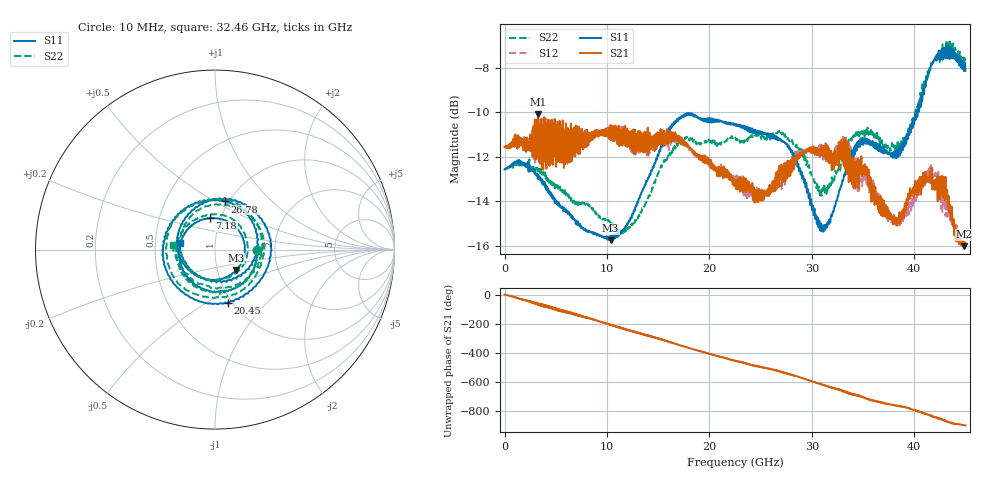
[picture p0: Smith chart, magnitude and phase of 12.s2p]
! 9/19/2025 2:51:32 PM
! C:\USERS\VECTORSTARUSER\DESKTOP\1942\12.S2P
! CHANNEL.1
! TR.MEASUREMENT
! CORRECTED.DATA
! RF.CORRECTION: FULL.TWO.PORT.CAL.PORT.1.2
! AVERAGING.OFF
! IF.BANDWIDTH: 1KHZ
! SWEEPTYPE:  FREQ.SWEEP(Linear)
! Reference Plane Port Info
! PORT:  PORT1  PORT2
! DISTANCE:  0  m  0  m
! TIME:  0  s  0  s
! PHASE.OFFSET:  0 °  0 °
! LOSS:  0  dB  0  dB
! REF.LOSS:  0  dB  0  dB
! REF.FREQ:  0  Hz  0  Hz
! Power Info
! POWER:  -10  dBm  -10  dBm
! EFF.POWER:  -10  dBm  -10  dBm
! SOURCE.ATTEN:  0  dB  0  dB
! TEST.ATTEN:  0  dB  0  dB
# GHZ S RI R 50.0
! FREQ.GHZ  S11RE  S11IM  S21RE  S21IM  S12RE  S12IM  S22RE  S22IM
!; PortSelection: Port_12
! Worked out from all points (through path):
!   1601 points, 10 MHz to 45 GHz, reference 50 ohm
!   highest |S21| = -10.10 dB at 3.272 GHz (marker M1); lowest = -16.0 dB at 44.86 GHz (marker M2)
!   group delay of S21, straight-line fit = 55.4 ps
!   lowest |S11| = -15.8 dB at 10.36 GHz (marker M3), VSWR 1.39, Z = 61.3 - j14.3 ohm
!   |S11| at or under -10 dB: start of sweep to 40.21 GHz; 40.25848 GHz to 40.34143 GHz (82.95 MHz wide, 0.206 % of centre)
!   |S22| runs from -15.5 to -6.8 dB; largest |S21 - S12| = 0.072
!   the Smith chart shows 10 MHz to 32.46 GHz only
!   S11 on the Smith chart (normalised r, x): 10 MHz: 1.62, -0.00; 7.18 GHz: 0.89, +0.33; 20.45 GHz: 0.96, -0.63; 26.78 GHz: 0.96, +0.56; 32.46 GHz: 0.67, +0.05
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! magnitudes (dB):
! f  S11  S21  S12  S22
! 10 MHz  -12.6  -11.6  -11.6  -12.6
! 3.272 GHz  -12.8  -10.1  -12.1  -12.6
! 7.18 GHz  -14.9  -10.8  -11.7  -14.1
! 7.518 GHz  -15.1  -11.5  -10.8  -14.1
! 10.36 GHz  -15.8  -10.6  -10.9  -15.0
! 12.49 GHz  -14.6  -11.2  -11.3  -15.1
! 15.03 GHz  -11.9  -11.1  -11.5  -12.7
! 17.25 GHz  -10.3  -11.3  -11.4  -11.3
! 20.45 GHz  -10.3  -12.4  -12.7  -11.3
! 22.5 GHz  -10.5  -13.2  -12.9  -11.2
! 25.23 GHz  -10.9  -13.7  -13.5  -11.2
! 26.78 GHz  -11.3  -13.4  -13.0  -10.9
! 30.01 GHz  -14.4  -11.6  -11.7  -12.9
! 31.19 GHz  -15.2  -11.5  -11.7  -13.4
! 32.46 GHz  -14.0  -12.1  -11.8  -12.6
! 34.62 GHz  -11.3  -12.4  -13.5  -11.1
! 37.52 GHz  -11.8  -14.4  -14.5  -11.7
! 39.01 GHz  -11.4  -14.7  -14.7  -11.5
! 41.57 GHz  -8.0  -13.2  -12.5  -8.1
! 43.31 GHz  -7.4  -14.3  -14.1  -6.8
! 44.86 GHz  -8.1  -16.0  -15.9  -7.7
! 45 GHz  -8.1  -15.9  -15.9  -7.6
